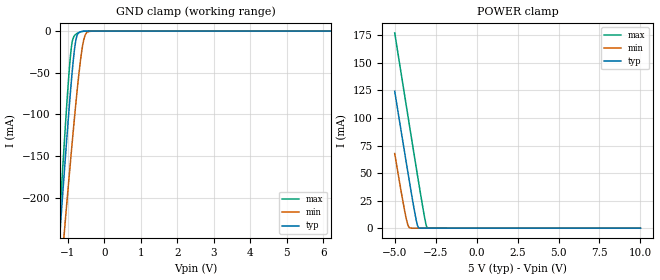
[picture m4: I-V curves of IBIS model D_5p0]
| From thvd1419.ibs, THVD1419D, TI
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|   D_5p0 Model
[Model]   D_5p0
Model_type   Input
Vinl = 0.8
Vinh = 2
|   typ   min   max
C_comp   2.237pF   2.186pF   2.332pF
| Where Nom  PVT is Nominal Process, 5.0V, 25C
|   Fast PVT is Strong Process,  5.5V, -40C
|   Slow PVT is Weak Process,   4.5V, 150C
[Voltage Range]   5   4.5   5.5
|Junction Temperature
[Temperature Range]   25   150   -40
[Power Clamp Reference]   5   4.5   5.5
[GND Clamp Reference]   0   0   0
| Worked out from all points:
|   GND clamp passes 1 mA (typ) near -0.66 V on its own axis
|   POWER clamp passes 1 mA (typ) near -3.57 V on its own axis
[GND Clamp]
|   Voltage   I(typ)   I(min)   I(max)
-5V       -2.702A    -2.362A    -3.144A
-1.235V   -254.9mA   -314mA     -234.4mA
-1.145V   -199.8mA   -267.4mA   -169.4mA
-1.07V    -154.7mA   -229mA     -117mA
-965mV    -94.16mA   -176.1mA   -49.96mA
-905mV    -61.98mA   -146.5mA   -21mA
-860mV    -40.13mA   -124.8mA   -9.488mA
-785mV    -12.66mA   -89.94mA   -4.069mA
-650mV    -835.5uA   -34.59mA   -894.9uA
-545mV    -147.3uA   -7.604mA   -141.3uA
-410mV    -13.38uA   -326.2uA   -9.602uA
10V       0A         0A         0A
[POWER Clamp]
|   Voltage   I(typ)   I(min)   I(max)
-5V       124.2mA    67.71mA    177.2mA
-4.385V   67.83mA    15.16mA    119.7mA
-4.265V   56.95mA    6.676mA    108.5mA
-4.175V   48.85mA    2.121mA    100.2mA
-4.07V    39.48mA    223uA      90.41mA
-3.785V   14.95mA    160.7nA    64.06mA
-3.605V   2.368mA    23.94nA    47.57mA
-3.515V   184.2uA    18.68nA    39.4mA
-3.155V   0A         3.524nA    8.204mA
-3.065V   0A         425.8pA    2.154mA
-3.005V   0A         0A         289.6uA
10V       0A         0A         0A
